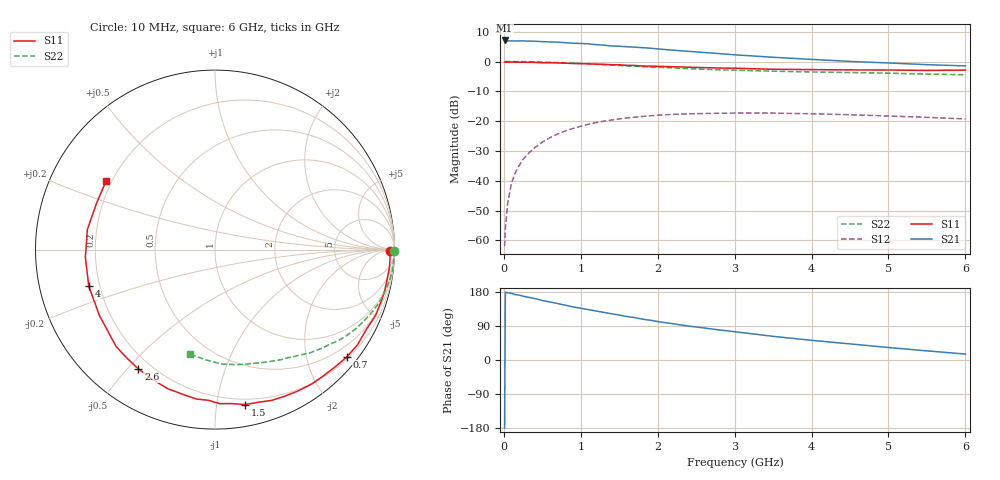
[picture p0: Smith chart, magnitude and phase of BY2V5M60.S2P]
! SIEMENS Small Signal Semiconductors
! BFY420
! Si NPN RF SIEGET Grounded Emitter Transistor in MICRO-X
! VCE = 2.5 V  IC = 0.6 mA
! Common Emitter S-Parameters:  October  1996
# GHz  S  MA  R  50
!  f  S11  S21  S12  S22
! GHz  MAG  ANG  MAG  ANG  MAG  ANG  MAG  ANG
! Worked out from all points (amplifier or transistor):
!   36 points, 10 MHz to 6 GHz, reference 50 ohm
!   highest |S21| = 7.1 dB at 10 MHz (marker M1)
!   |S21| within 3 dB of that: start of sweep to 2.077 GHz
!   unconditionally stable (mu >= 1): 4.725 GHz to end of sweep
!   at 250 MHz: K = 0.04, MSG = 19.9 dB, |S12| = -32.8 dB
!   at 1.4 GHz: K = 0.18, MSG = 12.4 dB, |S12| = -19.6 dB
!   at 6 GHz: K = 1.40, MAG = 5.1 dB, |S12| = -19.3 dB
!   S11 on the Smith chart (normalised r, x): 10 MHz: 68, -29; 700 MHz: 0.24, -2.81; 1.5 GHz: 0.16, -1.20; 2.6 GHz: 0.15, -0.54; 4 GHz: 0.16, -0.14; 6 GHz: 0.18, +0.28
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0.01  0.9754 -0.6  2.255 -179.3  0.0008 94.9  0.9996 -0.3
0.02  0.9735 -1.3  2.236 178.9  0.0016 82.2  0.9972 -0.5
0.05  0.9765 -2.7  2.222 177.3  0.0042 90.4  0.9991 -1.3
0.1  0.9772 -5.9  2.22 175.9  0.0092 87.0  0.9977 -2.7
0.15  0.974 -8.6  2.21 172.5  0.0137 83.3  0.9968 -4.0
0.25  0.9729 -14.0  2.218 168.6  0.0228 80.5  0.995 -6.6
0.4  0.967 -22.3  2.19 162.4  0.0358 76.0  0.985 -10.6
0.5  0.9531 -28.0  2.154 157.0  0.0443 72.8  0.9778 -13.2
0.7  0.9475 -39.0  2.108 148.9  0.0609 66.2  0.9592 -18.2
0.9  0.9271 -49.5  2.032 140.1  0.0756 58.9  0.9348 -22.9
1.1  0.9128 -59.9  1.976 132.9  0.0887 52.9  0.9101 -27.5
1.5  0.8793 -79.1  1.805 118.7  0.1088 41.3  0.8593 -35.6
1.8  0.8402 -92.6  1.709 107.8  0.1197 33.8  0.8209 -40.9
2.2  0.8184 -108.9  1.549 95.5  0.1301 24.6  0.781 -47.6
2.6  0.79 -122.7  1.418 84.6  0.1344 17.3  0.7419 -53.4
3  0.7714 -135.6  1.296 74.6  0.1363 10.8  0.7152 -59.1
3.5  0.7413 -150.3  1.178 62.4  0.1363 4.0  0.6883 -65.5
4  0.732 -163.9  1.085 51.9  0.1329 -1.4  0.6678 -72.1
4.5  0.7234 -176.7  1.003 42.5  0.128 -5.9  0.6533 -79.0
5  0.7197 171.1  0.945 33.0  0.1219 -8.8  0.6379 -87.0
5.5  0.7089 158.7  0.885 24.1  0.1157 -10.6  0.6164 -94.8
6  0.718 147.6  0.844 15.7  0.1088 -10.3  0.5993 -103.6
